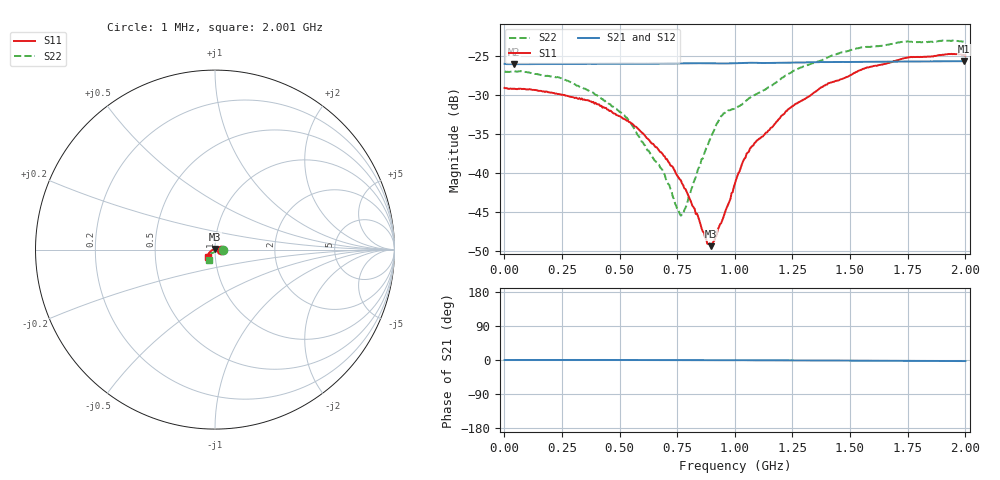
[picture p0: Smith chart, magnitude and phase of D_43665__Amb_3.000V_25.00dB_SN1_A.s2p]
! device id: 43665_
! dir: \\malibu\benchdata\1_engineers\tn_data\43665_75ohm\new\sparar\43665_\amb\3p000v\25p00db
! Serial: 1
! Insertion: A
! Temp: Amb
! VDD: 3.000V
! Attenuation Step: 25.00dB
! IDD: 1.451313e+00mA
! FILE NAME
! DATE 03-27-2009 08:39:30
! CORRECTED  DATA
#  Hz  S  RI  R  75
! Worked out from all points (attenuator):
!   401 points, 1 MHz to 2.001 GHz, reference 75 ohm
!   highest |S21| = -25.72 dB at 1.996 GHz (marker M1); lowest = -26.1 dB at 41 MHz (marker M2)
!   lowest |S11| = -49.4 dB at 896 MHz (marker M3), VSWR 1.01, Z = 74.7 + j0.424 ohm
!   |S11| at or under -10 dB: start of sweep to end of sweep
!   |S22| runs from -45.5 to -23.1 dB; largest |S21 - S12| = 0.00028
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1000000  0.0349 -0.000409  0.0497 -1.64e-05  0.0496 -0.00011  0.0446 -0.000255
4.1e7  0.0345 0.000639  0.0495 -4.35e-06  0.0495 3.55e-05  0.0446 0.000752
2.36e8  0.0316 0.00429  0.0496 7.11e-05  0.0496 0.000104  0.0404 0.00562
3.36e8  0.0294 0.00534  0.0496 7.17e-05  0.0497 9.37e-05  0.0343 0.0068
5.26e8  0.0208 0.00701  0.0498 -5.78e-05  0.0499 4.04e-06  0.0223 0.00426
6.71e8  0.0123 0.00646  0.0499 -2.91e-05  0.0499 2.19e-05  0.0112 -0.000122
7.16e8  0.00976 0.00614  0.05 -7.93e-05  0.05 -2.29e-06  0.0082 -0.0015
7.51e8  0.00776 0.00555  0.05 -0.000154  0.0501 -3.31e-05  0.00493 -0.00298
7.71e8  0.0066 0.0054  0.05 -0.000214  0.0501 -9.26e-05  0.00329 -0.00427
8.76e8  -0.000417 0.00372  0.0502 -0.000426  0.0502 -0.000319  -0.00465 -0.0136
8.96e8  -0.00185 0.00284  0.0501 -0.000482  0.0502 -0.000333  -0.00653 -0.0154
9.46e8  -0.00486 0.00105  0.05 -0.000494  0.05 -0.000329  -0.0138 -0.0188
1.001e9  -0.00852 0.000405  0.0502 -0.000308  0.0502 -0.000132  -0.0187 -0.0177
1.041e9  -0.0122 -0.000707  0.0504 -0.000381  0.0505 -0.000254  -0.0199 -0.0198
1.076e9  -0.0146 -0.00261  0.0505 -0.000634  0.0506 -0.000476  -0.0206 -0.0228
1.231e9  -0.0239 -0.0088  0.0506 -0.000781  0.0507 -0.000603  -0.0259 -0.034
1.336e9  -0.0288 -0.0138  0.0509 -0.000933  0.0511 -0.000777  -0.0292 -0.0407
1.546e9  -0.0376 -0.0255  0.0512 -0.00165  0.0514 -0.00147  -0.0333 -0.0537
1.671e9  -0.0395 -0.0315  0.0513 -0.00192  0.0515 -0.0018  -0.0339 -0.0568
1.756e9  -0.0407 -0.0367  0.0514 -0.00211  0.0516 -0.00204  -0.0331 -0.0604
1.996e9  -0.037 -0.0426  0.0517 -0.00255  0.0518 -0.00254  -0.0319 -0.061
2.001e9  -0.0371 -0.0423  0.0517 -0.00251  0.0517 -0.00255  -0.0321 -0.0606
